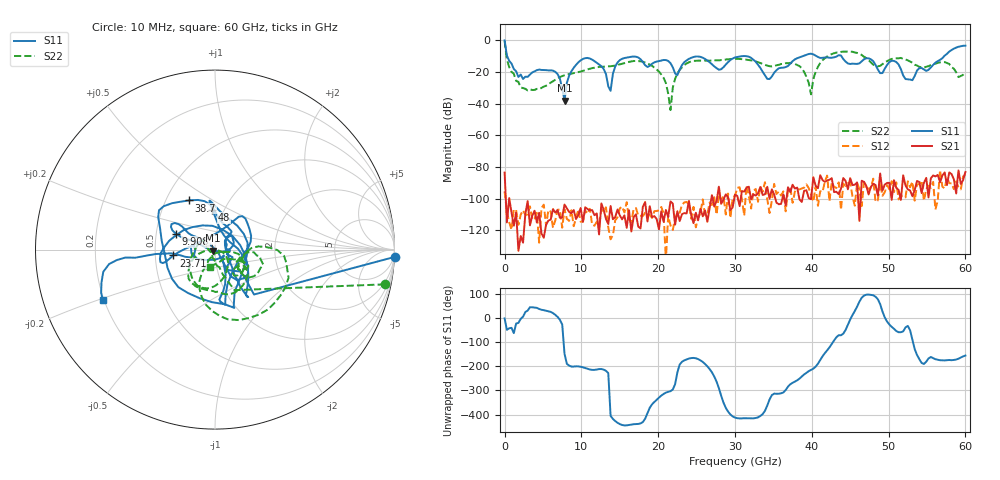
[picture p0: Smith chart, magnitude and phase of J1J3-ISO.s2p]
!Keysight Technologies,N5227A,US51270214,A.10.65.11
!Date: Thursday, October 15, 2020 08:08:22
!Correction: S11(Full 2 Port(1,2))
!S21(Full 2 Port(1,2))
!S12(Full 2 Port(1,2))
!S22(Full 2 Port(1,2))
!S2P File: Measurements: S11, S21, S12, S22:
# Hz S  dB  R 50
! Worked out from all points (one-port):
!   201 points, 10 MHz to 60 GHz, reference 50 ohm
!   lowest |S11| = -38.0 dB at 7.809 GHz (marker M1), VSWR 1.03, Z = 48.9 - j0.651 ohm
!   |S11| at or under -10 dB: 346.8 MHz to 30.83 GHz (30.48 GHz wide, 196 % of centre); 31.55 GHz to 38.8 GHz (7.247 GHz wide, 20.6 % of centre); 43.87 GHz to 57.22 GHz (13.35 GHz wide, 26.4 % of centre)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
!   S11 on the Smith chart (normalised r, x): 10 MHz: -1, -49; 9.908 GHz: 0.63, +0.12; 23.71 GHz: 0.62, -0.04; 38.7 GHz: 0.65, +0.40; 48 GHz: 0.88, +0.41; 60 GHz: 0.19, -0.21
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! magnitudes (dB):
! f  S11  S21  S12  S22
! 10 MHz  0.0  -83.5  -95.4  -0.3
! 2.11 GHz  -21.5  -123.6  -110.0  -29.7
! 6.609 GHz  -19.8  -108.8  -113.7  -24.9
! 7.809 GHz  -38.0  -103.7  -106.7  -22.0
! 9.908 GHz  -12.6  -105.9  -114.5  -19.7
! 10.21 GHz  -11.7  -114.7  -114.4  -19.2
! 13.81 GHz  -31.8  -104.6  -125.7  -16.3
! 15.01 GHz  -12.4  -110.5  -106.1  -15.1
! 20.11 GHz  -13.0  -119.4  -107.4  -19.7
! 21.61 GHz  -14.4  -101.7  -116.9  -44.0
! 22.21 GHz  -20.8  -116.5  -112.5  -24.3
! 23.71 GHz  -12.6  -109.3  -102.1  -14.5
! 30 GHz  -10.7  -97.4  -98.1  -11.6
! 34.5 GHz  -24.4  -100.0  -109.0  -16.2
! 38.7 GHz  -10.2  -102.1  -93.6  -17.5
! 39.9 GHz  -8.4  -100.3  -97.4  -34.0
! 40.2 GHz  -8.8  -86.4  -101.8  -24.4
! 43.2 GHz  -10.2  -95.6  -93.2  -7.6
! 48 GHz  -13.1  -90.6  -87.3  -15.3
! 50.1 GHz  -13.6  -90.0  -94.0  -12.3
! 53.1 GHz  -25.1  -98.4  -89.3  -14.1
! 60 GHz  -3.3  -83.1  -84.7  -19.9
